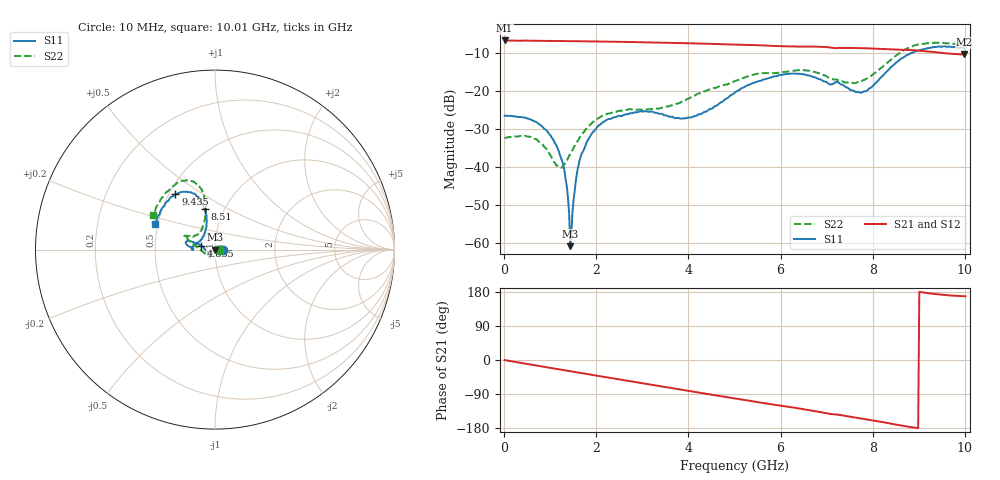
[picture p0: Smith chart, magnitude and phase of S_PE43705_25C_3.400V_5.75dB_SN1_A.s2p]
! Device ID: PE43705
! Serial: 1
! Insertion: A
! Impedance: 50 ohm
! Temp: 25C
! VDD: 3.400V
! Attenuation Step: 5.75dB
#  Hz  S  RI  R  50
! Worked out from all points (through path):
!   401 points, 10 MHz to 10.01 GHz, reference 50 ohm
!   highest |S21| = -6.81 dB at 10 MHz (marker M1); lowest = -10.5 dB at 9.985 GHz (marker M2)
!   group delay of S21, straight-line fit = 54.7 ps
!   lowest |S11| = -60.7 dB at 1.435 GHz (marker M3), VSWR 1.00, Z = 50.1 - j0.00967 ohm
!   |S11| at or under -10 dB: start of sweep to 8.857 GHz
!   |S22| runs from -40.1 to -7.4 dB; largest |S21 - S12| = 0.0041
!   S11 on the Smith chart (normalised r, x): 10 MHz: 1.10, -0.00; 4.835 GHz: 0.86, +0.04; 8.51 GHz: 0.81, +0.39; 9.435 GHz: 0.54, +0.39; 10.01 GHz: 0.48, +0.16
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1e7  0.0472 -8.42e-05  0.4564 -0.00214  0.457 -0.00208  0.0243 0.00013
6.6e8  0.0358 0.0174  0.439 -0.1078  0.4389 -0.1075  0.016 0.0172
1.06e9  0.0189 0.0135  0.4161 -0.1686  0.4163 -0.1685  0.00134 0.0125
1.285e9  0.00834 0.00634  0.4007 -0.2003  0.4008 -0.2002  -0.00855 0.00626
1.435e9  0.000913 -9.65e-05  0.3885 -0.2214  0.3886 -0.2211  -0.0151 0.00071
1.485e9  -0.00103 -0.00247  0.3842 -0.2281  0.3843 -0.228  -0.0166 -0.00157
1.585e9  -0.00615 -0.00619  0.3749 -0.241  0.3751 -0.241  -0.0208 -0.00536
1.685e9  -0.00992 -0.0114  0.3657 -0.2538  0.3658 -0.2538  -0.0253 -0.00951
1.885e9  -0.0177 -0.0196  0.3456 -0.2781  0.3458 -0.2778  -0.0329 -0.0168
2.21e9  -0.0247 -0.0326  0.3092 -0.3142  0.3094 -0.314  -0.0412 -0.0261
3.36e9  -0.0295 -0.0405  0.1555 -0.3982  0.156 -0.3978  -0.0537 -0.0231
4.085e9  -0.0436 -0.0137  0.0501 -0.4146  0.0506 -0.4145  -0.0851 -0.000557
4.835e9  -0.0765 0.0217  -0.0568 -0.4015  -0.0563 -0.4016  -0.1173 0.0284
5.01e9  -0.0902 0.0303  -0.0804 -0.3949  -0.0799 -0.395  -0.1292 0.0373
5.985e9  -0.1531 0.0482  -0.1931 -0.3318  -0.1913 -0.3324  -0.1588 0.0697
6.685e9  -0.1516 0.0225  -0.2614 -0.2743  -0.2617 -0.274  -0.1608 0.0773
7.76e9  -0.0714 0.0623  -0.3265 -0.1538  -0.3259 -0.1554  -0.0736 0.1125
8.36e9  -0.0474 0.1882  -0.3422 -0.0783  -0.341 -0.0799  -0.0527 0.2407
8.51e9  -0.0576 0.2272  -0.3413 -0.0564  -0.3404 -0.0594  -0.0586 0.2833
9.435e9  -0.2205 0.3085  -0.314 0.0386  -0.3129 0.0388  -0.2194 0.3643
9.985e9  -0.3276 0.1508  -0.2928 0.0602  -0.2937 0.0604  -0.3371 0.2053
1.001e10  -0.3353 0.1413  -0.2935 0.0615  -0.2947 0.0604  -0.345 0.1939
